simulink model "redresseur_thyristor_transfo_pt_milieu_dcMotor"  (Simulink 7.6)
settings: Solver=ode23tb  StartTime=0.0  StopTime=N  RelTol=1e-4
InitFcn:
  | clear all, close all, clc
  | N=15;
  | Couple=20;
  | ton=7;
  | toff=9;
StopFcn:
  | close all, clc
  | load Thyristor_dcMotor.mat
  | subplot 211
  | plot(x(1,:),x(2,:))
  | grid
  | axis([0 N -30 100])
  | title('Vitesse moteur')
  | xlabel('temps')
  | 
  | subplot 212
  | plot(x(1,:),x(3,:))
  | title('courant armature')
  | grid
  | xlabel('temps')
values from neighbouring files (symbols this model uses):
  A = [1+j -(1-j);1 -2/(1-j)]    [systeme_AX_B_phaseurs.m]
undefined symbols (not defined in the file or in its folder): constant, Torque
libraries: powerlib x8, simulink x4

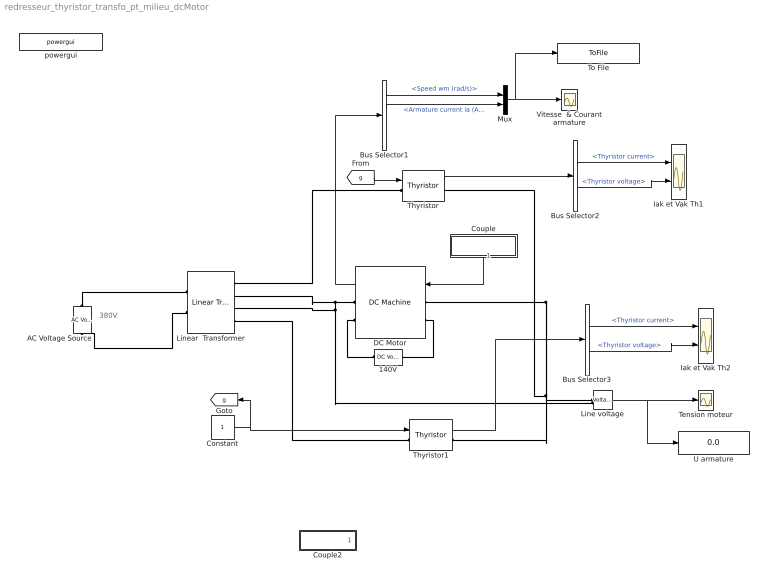
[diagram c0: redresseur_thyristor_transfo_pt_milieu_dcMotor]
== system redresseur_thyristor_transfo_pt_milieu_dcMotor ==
  note: 380V
  140V : powerlib/Electrical Sources/DC Voltage Source  DialogController=POWERSYS.PowerSysDialog  SystemSampleTime=-1  Amplitude=240  Measurements=None
  AC Voltage Source : powerlib/Electrical Sources/AC Voltage Source  DialogController=POWERSYS.PowerSysDialog  SystemSampleTime=-1  Amplitude=340  Phase=0  Frequency=60  SampleTime=0  Measurements=None
  Bus Selector1 : BusSelector  OutputSignals=Speed wm (rad/s),Armature current ia (A),Field current if (A),Electrical torque Te (n m)
  Bus Selector2 : BusSelector  OutputSignals=Thyristor current,Thyristor voltage
  Bus Selector3 : BusSelector  OutputSignals=Thyristor current,Thyristor voltage
  Constant : Constant
  Couple : Subsystem
  Couple2 : Subsystem
  DC Motor : powerlib/Machines/DC Machine  DialogController=POWERSYS.PowerSysDialog  SystemSampleTime=-1  PresetModel=No  MechanicalLoad=Torque TL  FieldType=Wound  ShowDetailedParameters=on  RLa="[ 0.1  0.012]"  RLf="[240  120]"  Laf=1.8  MachineConstant=Torque constant (N.m/A)  Ke=1.8  Kt=1.8  J=0.01  Bm=0  Tf=0  w0=0  Ifinit=1  TsPowergui=0  TsBlock=-1
  Iak et Vak Th1 : Scope  NumInputPorts=2
  Iak et Vak Th2 : Scope  NumInputPorts=2
  Line voltage : powerlib/Measurements/Voltage Measurement  Tag=PoWeRsYsTeMmEaSuReMeNt  DialogController=POWERSYS.PowerSysDialog  SystemSampleTime=-1  PhasorSimulation=off  OutputType=Magnitude  PSBequivalent=0
  Linear  Transformer : powerlib/Elements/Linear Transformer  DialogController=POWERSYS.PowerSysDialog  PhysicalDomain=powersysdomain  SubClassName=unknown  LeftPortType=p1  RightPortType=p1  LConnTagsString=a|b  RConnTagsString=A|B|C|D  UNITS=pu  NominalPower=[ 250e6 60 ]  winding1="[ 735e3  0.002  0.08 ]"  winding2="[ 315e3  0.002  0.08 ]"  ThreeWindings=on  winding3=[ 315e3 0.002 0.08 ]  RmLm=[ 500 500 ]  Measurements=None  DataType=off
  Mux : Mux  Inputs=2
  Tension moteur : Scope
  Thyristor : powerlib/Power Electronics/Thyristor  DialogController=POWERSYS.PowerSysDialog  SystemSampleTime=-1  Ron=0.001  Lon=0  Vf=0.8  IC=0  Rs=500  Cs=250e-9  Measurements=on
  Thyristor1 : powerlib/Power Electronics/Thyristor  DialogController=POWERSYS.PowerSysDialog  SystemSampleTime=-1  Ron=0.001  Lon=0  Vf=0.8  IC=0  Rs=500  Cs=250e-9  Measurements=on
  To File : ToFile  Filename=Thyristor_dcMotor  MatrixName=x
  U armature : Display
  Vitesse  & Courant armature : Scope
  powergui : powerlib/powergui  Priority=1  SystemSampleTime=-1  SimulationMode=Continuous  SampleTime=50e-6  frequency=60  SPID=off  DisableSnubberDevices=off  DisableRonSwitches=off  DisableVfSwitches=off  SwTol=0  Interpol=off  frequencyindice=0  echomessages=off  HookPort=off  DisplayEquations=off  FunctionMessages=off  EnableUseOfTLC=off  x0status=blocks  RestoreLinks=warning  ResistiveCurrentMeasurement=off  Ylog=off  Xlog=on  ShowGrid=off  save=off  variable=ZData  ZoomFFT=off  StartTime=0.0  cycles=1  DisplayStyle=1  fundamental=60  FreqAxis=off  MaxFrequency=1000  frequencyindicesteady=1  display=off  methode=off
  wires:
  Mux/1 -> Vitesse  & Courant armature/1, To File/1
  Constant/1 -> Thyristor1/1, [g]
  [g] -> Thyristor/1
  Bus Selector1/1 -> Mux/1  "<Speed wm (rad/s)>"
  Couple/1(Out1) -> DC Motor/1
  DC Motor/1 -> Bus Selector1/1
  Line voltage/1 -> Tension moteur/1, U armature/1
  Thyristor/1 -> Bus Selector2/1
  Bus Selector2/1 -> Iak et Vak Th1/1  "<Thyristor current>"
  Bus Selector2/2 -> Iak et Vak Th1/2  "<Thyristor voltage>"
  Thyristor1/1 -> Bus Selector3/1
  Bus Selector3/1 -> Iak et Vak Th2/1  "<Thyristor current>"
  Bus Selector3/2 -> Iak et Vak Th2/2  "<Thyristor voltage>"
  Bus Selector1/2 -> Mux/2  "<Armature current ia (A)>"
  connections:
  Linear  Transformer/LConn2 -- AC Voltage Source/LConn1
  AC Voltage Source/RConn1 -- Linear  Transformer/LConn1
  Linear  Transformer/RConn4 -- Thyristor1/LConn1
  Thyristor/LConn1 -- Linear  Transformer/RConn1
  Thyristor/RConn1 -- DC Motor/LConn1 -- Thyristor1/RConn1 -- Line voltage/LConn1
  140V/LConn1 -- DC Motor/RConn2
  140V/RConn1 -- DC Motor/LConn2
  DC Motor/RConn1 -- Linear  Transformer/RConn3 -- Line voltage/LConn2 -- Linear  Transformer/RConn2

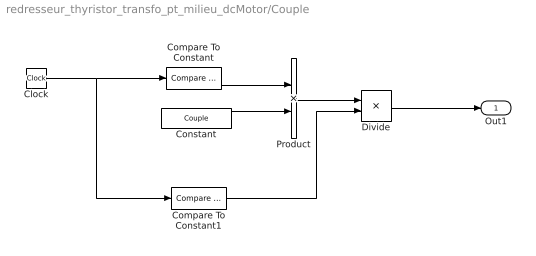
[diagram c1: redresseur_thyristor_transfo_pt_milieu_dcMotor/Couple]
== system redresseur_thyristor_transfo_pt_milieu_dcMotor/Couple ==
  Clock : Clock
  Compare To Constant : simulink/Logic and Bit Operations/Compare To Constant  SystemSampleTime=-1  relop=>=  const=ton  LogicOutDataTypeMode=uint8
  Compare To Constant1 : simulink/Logic and Bit Operations/Compare To Constant  SystemSampleTime=-1  relop=<=  const=toff  LogicOutDataTypeMode=uint8
  Constant : Constant  Value=Couple
  Divide : Product  Inputs=**
  Product : Product
  Out1 : Outport
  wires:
  Divide/1 -> Out1/1
  Compare To Constant1/1 -> Divide/2
  Product/1 -> Divide/1
  Constant/1 -> Product/2
  Compare To Constant/1 -> Product/1
  Clock/1 -> Compare To Constant1/1, Compare To Constant/1

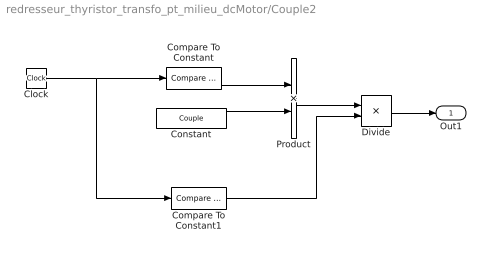
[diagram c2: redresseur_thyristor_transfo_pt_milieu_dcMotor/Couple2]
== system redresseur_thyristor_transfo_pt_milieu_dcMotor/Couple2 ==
  Clock : Clock
  Compare To Constant : simulink/Logic and Bit Operations/Compare To Constant  SystemSampleTime=-1  relop=>=  const=ton  LogicOutDataTypeMode=uint8
  Compare To Constant1 : simulink/Logic and Bit Operations/Compare To Constant  SystemSampleTime=-1  relop=>=  const=toff  LogicOutDataTypeMode=uint8
  Constant : Constant  Value=Couple
  Divide : Product  Inputs=**
  Product : Product
  Out1 : Outport
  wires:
  Divide/1 -> Out1/1
  Compare To Constant1/1 -> Divide/2
  Product/1 -> Divide/1
  Constant/1 -> Product/2
  Compare To Constant/1 -> Product/1
  Clock/1 -> Compare To Constant1/1, Compare To Constant/1
